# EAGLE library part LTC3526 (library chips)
Low power boost converter IC
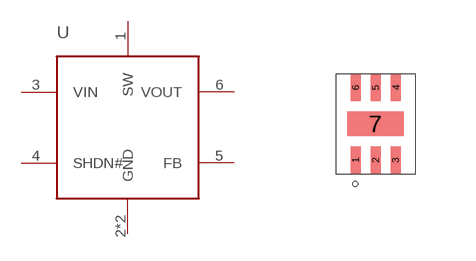
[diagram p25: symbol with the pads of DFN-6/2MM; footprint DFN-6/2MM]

Designator prefix -

## LTC3526 (DIGIKEY: LTC3526LEDC#TRMPBFCT-ND)  [DFN-6/2MM]
1  SW
2  GND
3  VIN
4  SHDN#
5  FB
6  VOUT
7  GND

## Footprint DFN-6/2MM (pad centres in mm)
smd 0.25 x 0.675: 1 -0.5,-0.91; 2 0,-0.91; 3 0.5,-0.91; 4 0.51,0.91; 5 0,0.91; 6 -0.5,0.91
smd 1.42 x 0.61: 7 0,0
